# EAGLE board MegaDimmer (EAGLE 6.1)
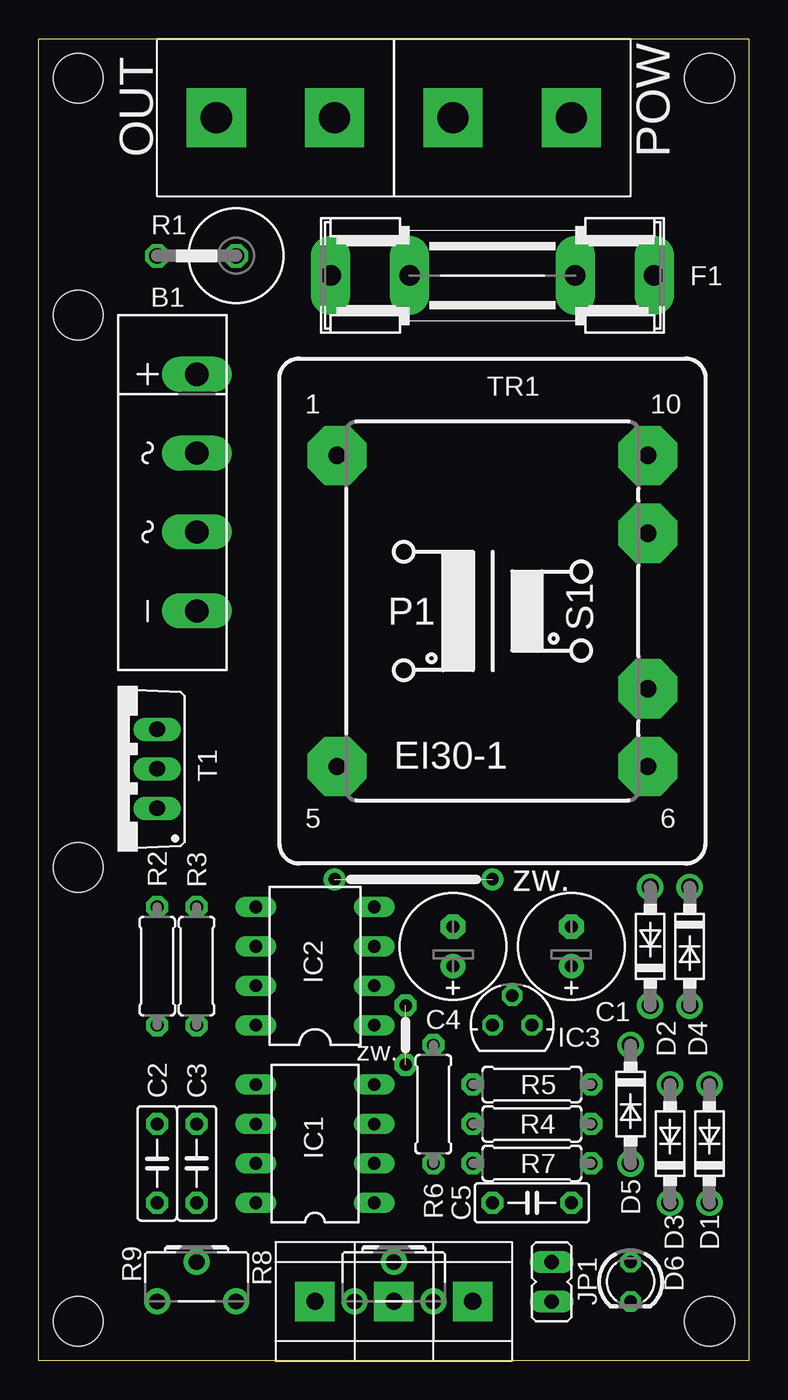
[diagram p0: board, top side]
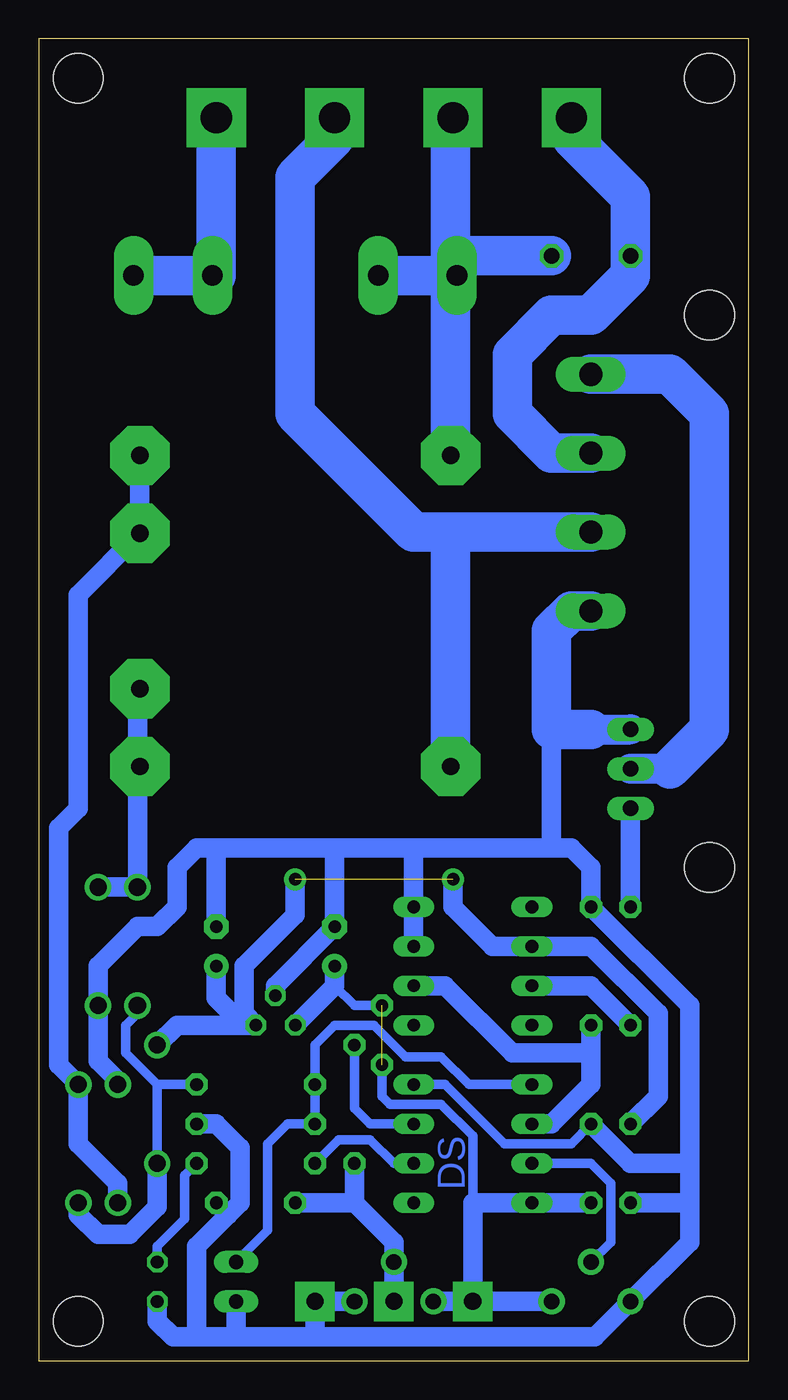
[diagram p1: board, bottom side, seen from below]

Size 45.72 x 85.09 mm. Coordinates in mm from the lower left corner, seen from the top.
Outline: 0,85.09 45.72,85.09 45.72,0 0,0 0,85.09
Copper layers (1*16): Top 0.035mm / dielectric 1.5mm / Bottom 0.035mm
Design rules: minimum track width 10mil, minimum drill 24mil, track to track 8mil, track to pad 8mil, pad to pad 8mil, via to via 8mil, smd to smd 8mil, copper to edge 40mil, drill to drill 8mil, minimum pad ring 10mil, minimum via ring 8mil, stop-mask expansion 4mil, vias tented up to drill 0mil, thermal gap 10mil
Holes 3.2 mm at 2.54,82.55 2.54,67.31 43.18,82.55 2.54,2.54 43.18,2.54 2.54,31.75

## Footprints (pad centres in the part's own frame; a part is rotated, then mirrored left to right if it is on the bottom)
FBU4 = drill 1.499 long: + 7.62,-1.54; - -7.62,-1.54; AC1 2.54,-1.54; AC2 -2.54,-1.54
E2,5-7 = drill 0.813 pad 1.6: + -1.27,0 | drill 0.813 pad 1.6 octagon: - 1.27,0
C050-025X075 = drill 0.813 pad 1.422 octagon: 1 -2.54,0; 2 2.54,0
ARK500/2 = drill 1.1 pad 2.54 square: 1 -2.54,0; 2 2.54,0
DO41-7.6 = drill 1.1 pad 1.7: A 3.81,0; C -3.81,0
LED3MM = drill 0.813 octagon: A -1.27,0; K 1.27,0
SHK20L = drill 1.321 pad 2.54 long: 1A -10.414,0; 1B -5.334,0; 2A 10.414,0; 2B 5.334,0
DIL08 = drill 0.813 long: 1 -3.81,-3.81; 2 -1.27,-3.81; 3 1.27,-3.81; 4 3.81,-3.81; 5 3.81,3.81; 6 1.27,3.81; 7 -1.27,3.81; 8 -3.81,3.81
78LXX = drill 0.813 octagon: GND 0,1.905; IN 1.27,0; OUT -1.27,0
JP1 = drill 0.914 long: 1 0,-1.27; 2 0,1.27
ARK2/750 = drill 2 pad 3.81 square: 1 -3.81,0; 2 3.81,0
0617V = drill 1.016 octagon: 1 -2.54,0; 2 2.54,0
0207/7 = drill 0.813 pad 1.422 octagon: 1 -3.81,0; 2 3.81,0
CA6H = drill 1.016 pad 1.676: A -2.54,0; E 2.54,0; S 0,2.54
TO220BV = drill 1.016 long: D 0,-2.54; G -2.54,-2.54; S 2.54,-2.54
EI30-1 = drill 1.118 pad 3.81 octagon: 1 -10.008,10.008; 5 -10.008,-10.008; 6 10.008,-10.008; 7 10.008,-5.004; 9 10.008,5.004; 10 10.008,10.008

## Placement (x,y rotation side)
B1  [FBU4]  8.64,55.88 90 top
C1  100uF/25V  [E2,5-7]  34.29,26.67 90 top
C2  100nF  [C050-025X075]  7.62,12.7 270 top
C3  100nF  [C050-025X075]  10.16,12.7 90 top
C4  100uF/25V  [E2,5-7]  26.67,26.67 90 top
C5  100nF  [C050-025X075]  31.75,10.16 0 top
CON1  [ARK500/2]  25.4,3.81 0 top
CON3  [ARK500/2]  20.32,3.81 0 top
D1  [DO41-7.6]  43.18,13.97 90 top
D2  [DO41-7.6]  39.37,26.67 90 top
D3  [DO41-7.6]  40.64,13.97 90 top
D4  [DO41-7.6]  41.91,26.67 270 top
D5  [DO41-7.6]  38.1,16.51 270 top
D6  LED  [LED3MM]  38.1,5.08 270 top
F1  [SHK20L]  29.21,69.85 180 top
IC1  ATTINY25  [DIL08]  17.78,13.97 90 top
IC2  MC33152  [DIL08]  17.78,25.4 90 top
IC3  78L05  [78LXX]  30.48,21.59 0 top
JP1  [JP1]  33.02,5.08 0 top
OUT  ARK2  [ARK2/750]  15.24,80.01 180 top
POW  ARK2  [ARK2/750]  30.48,80.01 0 top
R1  100k  [0617V]  10.16,71.12 180 top
R2  100R  [0207/7]  7.62,25.4 90 top
R3  2.4k  [0207/7]  10.16,25.4 270 top
R4  22k  [0207/7]  31.75,15.24 180 top
R5  22k  [0207/7]  31.75,17.78 0 top
R6  2.4k  [0207/7]  25.4,16.51 270 top
R7  2.4k  [0207/7]  31.75,12.7 0 top
R8  50k  [CA6H]  22.86,3.81 0 top
R9  50k  [CA6H]  10.16,3.81 0 top
T1  P4NK60  [TO220BV]  5.08,38.1 90 top
TR1  [EI30-1]  29.21,48.26 0 top

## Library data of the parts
B1 = rectifier
C1-C5 R1-R7 = rcl
CON1 CON3 = DS
D1-D5 = diode
D6 = led
F1 = fuse; OC_FARNELL: unknown; OC_NEWARK: unknown
IC1 = avr-7
IC2 = ic-package
IC3 = v-reg
JP1 = jumper
OUT POW = dimmer
R8 R9 = pot
T1 = transistor-power
TR1 = trafo

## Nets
AC1: F1.2A OUT.1 R1.1 TR1.1
AC2: B1.AC2 POW.1 TR1.5
DRV: IC1.6 IC2.2 R3.2
GND: B1.- C1.- C2.2 C3.2 C4.- C5.2 CON1.2 D3.A D4.A D6.K IC1.4 IC2.3 IC2.4 IC3.GND JP1.1 R3.1 R4.1 R8.E R9.A T1.S
LED: IC1.2 R7.1
N$1: F1.1A POW.2
N$2: C5.1 CON1.1 CON3.2 R6.2 R8.S
N$3: B1.AC1 OUT.2 R1.2
N$4: B1.+ T1.D
N$6: R2.2 T1.G
N$7: IC2.7 R2.1
N$8: D1.A D3.C TR1.9
N$9: D2.A D4.C TR1.7
N$15: D6.A R7.2
PH: IC1.5 JP1.2 R4.2 R5.1
PHS: D1.C D2.C D5.A R5.2
VCC: C1.+ C2.1 D5.C IC2.6 IC3.IN
VDD: C3.1 C4.+ CON3.1 IC1.8 IC3.OUT R8.A R9.E
VR1: IC1.3 R6.1
VR2: IC1.7 R9.S

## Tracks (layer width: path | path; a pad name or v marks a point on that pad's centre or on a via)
AC1
  Bottom 2.54: TR1.1 19.2,69.85 | 19.2,69.85 19.2,70.87 | 19.2,70.87 19.2,79.86 OUT.1 | 19.2,69.85 F1.2A 23.88,69.85 | R1.1 18.95,71.12 19.2,70.87
AC2
  Bottom 2.54: POW.1 26.67,78.74 29.21,76.2 29.21,60.96 21.59,53.34 21.34,53.34 19.56,53.34 | TR1.5 19.2,52.98 19.56,53.34 | B1.AC2 19.56,53.34
DRV
  Bottom 1.27: IC2.2 19.56,24.13 15.24,19.81 10.16,19.81 | IC1.6 12.7,15.24 10.16,17.78 10.16,19.81 | R3.2 10.16,19.81
GND
  Bottom 0.61: C3.2 11.43,13.97 15.75,13.97 19.56,17.78 IC1.4
  Bottom 1.27: 21.59,33.02 IC2.4 IC2.3 | 12.7,33.02 12.7,40.89 | C1.- 34.29,33.02 | D3.A 40.64,18.03 41.91,19.3 D4.A 41.91,25.4 39.37,27.94 38.1,27.94 36.83,29.21 36.83,31.75 35.56,33.02 34.29,33.02 | 3.81,12.7 3.81,22.86 R3.1 10.16,31.75 11.43,33.02 12.7,33.02 | 3.81,12.7 3.81,10.16 | 3.81,10.16 3.81,7.62 R9.A 9.91,1.52 27.94,1.52 | 27.94,1.52 33.02,1.52 | 33.02,1.52 35.56,1.52 | 35.56,1.52 37.08,1.52 38.1,2.54 D6.K | C2.2 3.81,10.16 | 21.59,33.02 12.7,33.02 | 34.29,33.02 26.42,33.02 | 26.42,33.02 21.59,33.02 | 26.42,33.02 26.67,32.77 C4.- 30.48,24.13 IC3.GND | JP1.1 33.02,1.52 | C3.2 7.62,12.7 3.81,12.7 | R8.E CON1.2 27.94,1.52 | R4.1 34.29,15.24 32.77,13.72 32.77,10.16 33.53,9.4 | 33.53,9.4 35.56,7.37 35.56,1.52 | C5.2 33.53,9.4
  Bottom 1.93: 10.16,40.64 T1.S
  Bottom 2.54: B1.- 11.43,48.26 12.7,46.99 12.7,40.89 12.7,40.64 10.16,40.64
LED
  Bottom 0.61: R7.1 26.42,14.22 24.38,14.22 22.86,12.7 IC1.2
N$1
  Bottom 2.54: POW.2 34.29,69.85 F1.1A
N$2
  Bottom 1.27: CON1.1 R8.S 22.86,7.62 25.4,10.16 | 25.4,10.16 R6.2 | C5.1 25.4,10.16
N$3
  Bottom 2.54: OUT.2 11.43,78.74 7.62,74.93 R1.2 7.62,69.85 10.16,67.31 12.7,67.31 15.24,64.77 15.24,60.96 12.7,58.42 B1.AC1
N$4
  Bottom 1.93: 5.08,38.1 T1.D
  Bottom 2.54: B1.+ 5.08,63.5 2.54,60.96 2.54,40.64 5.08,38.1
N$6
  Bottom 1.27: R2.2 T1.G
N$7
  Bottom 1.27: IC2.7 10.16,24.13 R2.1
N$8
  Bottom 1.27: 39.37,58.42 39.22,58.27 TR1.9 43.18,49.3 43.18,35.56 44.45,34.29 44.45,19.05 D1.A 43.18,13.97 40.64,11.43 D3.C
N$9
  Bottom 1.27: TR1.7 39.37,43.1 D2.A D4.C
N$15
  Bottom 0.61: D6.A 38.1,7.37 36.32,9.14 36.32,11.94 R7.2
PH
  Bottom 0.61: JP1.2 30.99,8.38 30.99,13.97 29.72,15.24 R4.2 R5.1 27.94,20.32 26.67,21.59 24.13,21.59 22.1,19.56 19.81,19.56 18.03,17.78 IC1.5
PHS
  Bottom 0.61: 38.1,17.78 D5.A | D2.C 39.37,22.35 40.13,21.59 40.13,19.81 38.1,17.78 | R5.2 38.1,17.78
  Bottom 1.27: D5.A 38.1,9.91 39.88,8.13 41.91,8.13 43.18,9.4 D1.C
VCC  (via drill 0.8 pad 1.42)  (1 unrouted)
  Bottom 1.27: 32.51,21.59 IC3.IN 32.51,22.35 32.51,25.4 29.21,28.7 v29.21,30.99 | 32.51,21.59 36.83,21.59 D5.C | C2.1 5.84,17.02 5.84,22.35 10.16,26.67 IC2.6 16.51,26.67 19.05,29.21 v19.05,30.99 | C1.+ 34.29,23.37 32.51,21.59
VDD  (via drill 0.8 pad 1.42)  (1 unrouted)
  Bottom 0.61: 17.78,10.16 17.78,14.48 19.81,16.51 23.11,16.51 23.62,17.02 v23.62,19.05 | 28.96,21.84 IC3.OUT | v23.62,22.86 25.4,22.86 26.67,24.13
  Bottom 1.27: CON3.1 R9.E | CON3.1 17.78,10.16 IC1.8 C3.1 | C4.+ 26.67,24.13 IC3.OUT | R8.A CON3.1
VR1
  Bottom 0.61: IC1.3 24.38,15.24 25.4,16.26 R6.1
VR2
  Bottom 0.61: IC1.7 10.16,12.7 8.89,11.43 8.89,7.62 R9.S

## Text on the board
Bottom: DS
tPlace: zw. | zw.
